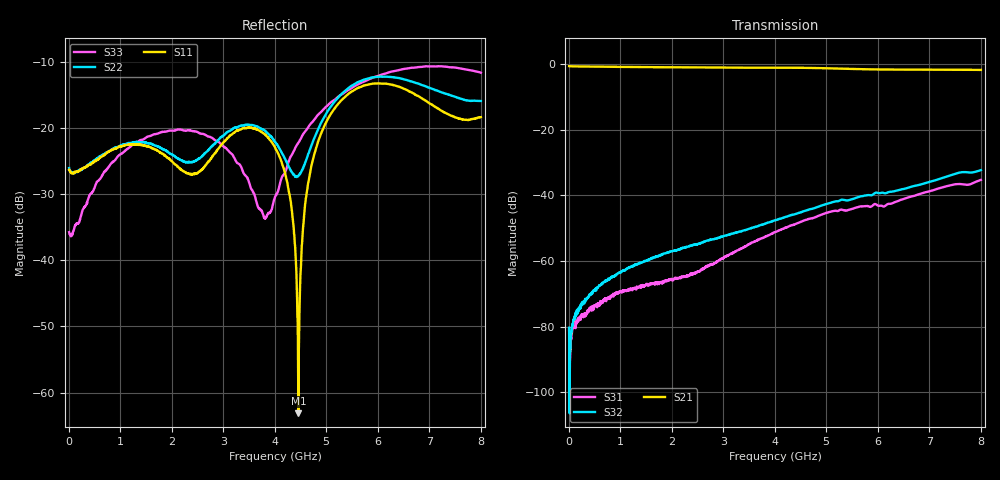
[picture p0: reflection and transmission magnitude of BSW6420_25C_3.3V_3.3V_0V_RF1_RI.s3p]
! Product: BSW6420
! Temp: 25C
! VDD: 3.300
! Control_Hi: 3.300
! Control_Lo: 0.000
! Logic State: RF1
! Port 1: RFC
! Port 2: RF1
! Port 3: RF2
! V1 = 0.00
! V2 = 3.30
! V3 = 0.00
! V4 = 0.00
# Hz S  RI  R 50
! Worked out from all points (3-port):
!   1601 points, 5 MHz to 8.005 GHz, reference 50 ohm
!   strongest paths, dB at 5 MHz, 2.005 GHz, 4.005 GHz, 6.005 GHz, 8.005 GHz:
!     S21: -0.6, -0.9, -1.1, -1.6, -1.8
!     S32: -80.3, -57.0, -47.6, -39.2, -32.3
!     S31: -80.5, -65.8, -51.1, -43.1, -35.3
!   lowest |S11| = -63.1 dB at 4.46 GHz (marker M1), VSWR 1.00, Z = 50 + j0.0673 ohm
!   |S11| at or under -10 dB: start of sweep to end of sweep
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5000000  0.0481 -0.00309  0.9327 -0.0118  5e-05 -3.03e-05
         0.9323 -0.0113  0.0496 -0.00341  4.44e-05 -3.67e-05
         5.68e-05 -7.58e-05  5.11e-05 -8.18e-05  0.0162 -0.00126
8.8e8  -0.0488 -0.0494  0.0161 -0.9115  0.000303 3.71e-06
       0.0159 -0.9114  -0.0502 -0.0485  0.000592 9.26e-05
       0.000314 2.54e-06  0.000573 0.000103  -0.0433 -0.0358
1.76e9  -0.0503 0.0425  -0.898 -0.046  0.000282 -0.000382
        -0.898 -0.0462  -0.0545 0.0465  0.000739 -0.000948
        0.000276 -0.000378  0.000726 -0.00096  -0.0733 0.055
2.775e9  -0.0417 0.0427  0.1354 0.8809  -0.000167 -0.000892
         0.1353 0.881  -0.0339 0.0635  -0.0014 -0.00162
         -0.000163 -0.000887  -0.00139 -0.00162  0.0406 0.074
4.005e9  0.0524 0.0483  0.6567 -0.5894  -0.00266 0.000763
         0.6566 -0.5897  0.0775 0.0105  -0.00284 0.00307
         -0.00267 0.000748  -0.00282 0.00309  -0.0257 -0.0157
4.46e9  0.000183 0.000673  0.0311 -0.8798  -0.00193 0.00332
        0.0311 -0.8798  -0.0095 -0.0425  -0.000272 0.0054
        -0.00193 0.0033  -0.000269 0.00539  -0.0636 0.0436
4.895e9  -0.0623 0.0643  -0.5855 -0.644  0.00117 0.00491
         -0.5856 -0.6439  -0.0998 0.0412  0.00418 0.00556
         0.00121 0.00489  0.00418 0.00556  -0.0363 0.1261
6.26e9  0.2119 0.00161  -0.0135 0.8279  0.00424 -0.00619
        -0.0132 0.8275  0.2325 0.0667  0.00215 -0.0112
        0.00421 -0.0062  0.00213 -0.0112  0.2649 -0.0201
7.14e9  -0.0273 -0.1398  0.8242 0.0285  -0.0092 -0.00845
        0.824 0.0282  0.0946 -0.1668  -0.0161 -0.00628
        -0.00919 -0.00842  -0.0161 -0.00627  0.0597 -0.285
8.005e9  -0.0968 0.0716  0.0451 -0.8165  -0.013 0.0114
         0.0447 -0.8162  -0.1183 -0.1072  -0.00939 0.0224
         -0.0129 0.0115  -0.00941 0.0224  -0.2439 -0.0925
